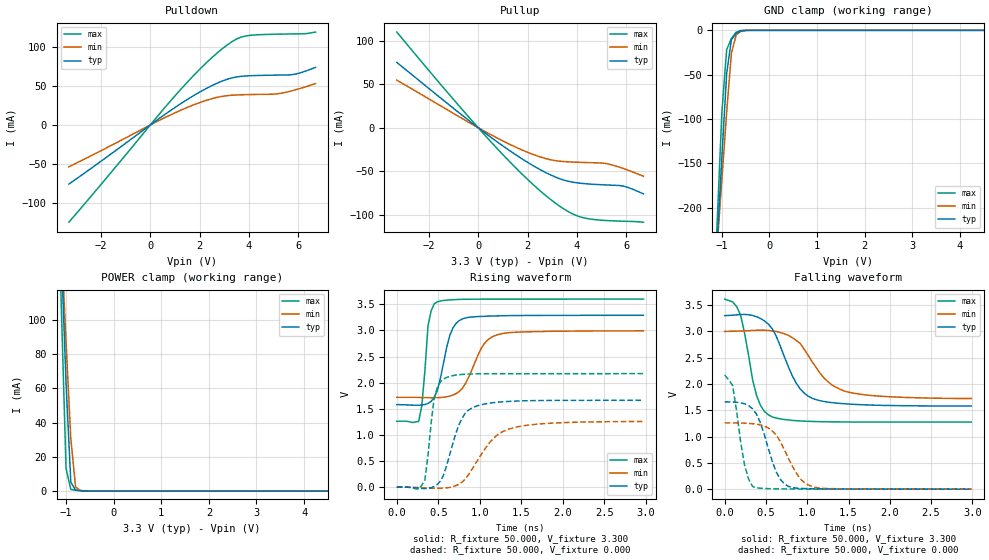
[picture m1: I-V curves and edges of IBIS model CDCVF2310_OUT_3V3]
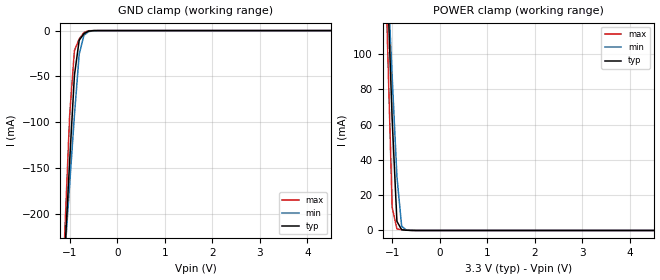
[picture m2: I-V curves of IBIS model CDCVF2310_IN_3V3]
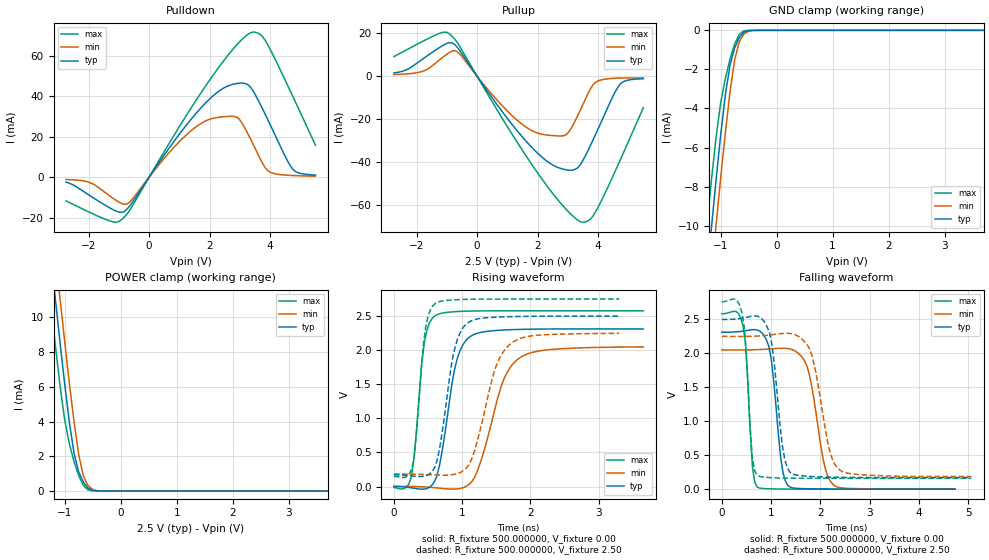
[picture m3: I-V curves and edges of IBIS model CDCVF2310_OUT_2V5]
|   TEXAS INSTRUMENTS INCORPORATED
|   CLOCK DISTRIBUTION CIRCUITS
|   IBIS Model of CDCVF2310
|   2.5-V TO 3.3-V High Performance Clock Buffer
|   24-pin (PW) Package
[IBIS Ver]   3.2
[File Name]   scac026c.ibs
[File Rev]   2.2 (10)
[Date]   12/15/2007
[Source]   File originated at Texas Instruments, Inc.
[Notes]   The following is an IBIS list for the CDCVF2310.
|   - All test data contained in this file are derived from
|   hspice(tm) simulations.
|   - File created by Gerd Baumann, HPA-Product Engineering.
|   07: added V-T tables,
|   08: corrected C_comp, revised clamp current
|   09: added R_load to ramp and corrected ramp rate
|   10: added Models for 2.5V VCC
|   (by Christian Schmoeller, 15-Dec-2007)
[Disclaimer] Property of Texas Instruments Incorporated.  Unauthorized
   reproduction and/or distribution is strictly prohibited.
   This product is protected under copyright law.
   Created 2000, (C) Copyright 2000, Texas Instruments Inc.,
   All Rights Reserved
   UNLESS THERE IS A SIGNED, WRITTEN AGREEMENT TO THE
   CONTRARY, TEXAS INSTRUMENTS ("TI") IS PROVIDING THE IBIS
   MODELS "AS IS" AND WITHOUT ANY WARRANTY, EXPRESSED OR
   IMPLIED.  TI assumes no liability for:
   1) the accuracy of the IBIS models provided to your
   company;
   2) the proper functioning of these IBIS models in your
   design or for any resulting applications; or
   3) infringement of patents, copyrights or intellectual
   property rights resulting from your use of these IBIS
   models.
   TI provides IBIS Models as a service to our customers.
   You and your company shall not distribute, sell or give
   these models to anyone else without prior written
   permission from TI.
   TI reserves the right to make changes to our products or
   to discontinue any semiconductor product or service
   without notice, and advises our customers to obtain the
   latest version of relevant information to verify, before
   placing orders, that the information being relied on is
   current.
   Please be aware that your receipt and use of the IBIS
   information provided shall serve as acceptance of these
   terms and conditions.  If you do not accept these terms,
   you should return or destroy the IBIS models and any
   other accompanying information immediately.
[Component]   CDCVF2310(High_Performance_Clock_Buffer)
[Manufacturer]  Texas Instruments, Inc.
[Package]
|   typ   min   max
R_pkg   0.034   0.031   0.040
L_pkg   2.71n   2.07n   3.51n
C_pkg   0.37p   0.24p   0.48p
[Pin]   signal_name   model_name   R_pin   L_pin   C_pin
 1   GND   GND   0.035   3.51n   0.48p
 2   VCC   POWER   0.040   3.26n   0.47p
 3   1Y0   CDCVF2310_OUT   0.035   2.96n   0.42p
 4   1Y1   CDCVF2310_OUT   0.031   2.33n   0.32p
 5   1Y2   CDCVF2310_OUT   0.032   2.14n   0.26p
 6   GND   GND   0.031   2.07n   0.24p
 7   GND   GND   0.031   2.07n   0.24p
 8   1Y3   CDCVF2310_OUT   0.032   2.14n   0.26p
 9   1Y4   CDCVF2310_OUT   0.031   2.33n   0.32p
10   VCC   POWER   0.035   2.96n   0.42p
11   1G   CDCVF2310_IN   0.040   3.26n   0.47p
12   2Y4   CDCVF2310_OUT   0.035   3.51n   0.48p
13   2G   CDCVF2310_IN   0.035   3.51n   0.48p
14   VCC   POWER   0.040   3.26n   0.47p
15   VCC   POWER   0.035   2.96n   0.42p
16   2Y3   CDCVF2310_OUT   0.031   2.33n   0.32p
17   2Y2   CDCVF2310_OUT   0.032   2.14n   0.26p
18   GND   GND   0.031   2.07n   0.24p
19   GND   GND   0.031   2.07n   0.24p
20   2Y1   CDCVF2310_OUT   0.032   2.14n   0.26p
21   2Y0   CDCVF2310_OUT   0.031   2.33n   0.32p
22   VCC   POWER   0.035   2.96n   0.42p
23   VCC   POWER   0.040   3.26n   0.47p
24   CLK   CDCVF2310_IN   0.035   3.51n   0.48p
[Model Selector]   CDCVF2310_IN
CDCVF2310_IN_2V5   Model for 2.5V VCC
CDCVF2310_IN_3V3   Model for 3.3V VCC
[Model Selector]   CDCVF2310_OUT
CDCVF2310_OUT_2V5   Model for 2.5V VCC
CDCVF2310_OUT_3V3   Model for 3.3V VCC
| Models and submodels in the file (4): CDCVF2310_OUT_3V3 (Output), CDCVF2310_IN_3V3 (Input), CDCVF2310_OUT_2V5 (Output), CDCVF2310_IN_2V5 (Input)
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|   Model CDCVF2510_OUT
[Model]   CDCVF2310_OUT_3V3
Model_type   Output
Polarity   Non-Inverting
Enable   Active-High
Vmeas = 1.65V   |Vref for timing measurements.
Cref = 25pF   |load capacitance for timing spec.
Rref = 500   |500 Ohm to GND.
Vref = 0   |Timing specification test load voltage; GND
| variable   typ   min   max
C_comp   2.4pF   NA   NA
[Temperature Range]   40   85   -40
[Voltage range]   3.3   3.0   3.6
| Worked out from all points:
|   slope of the pulldown table from 0 to 0.495 V, typ, clamps not added: 43.4 ohm
|   slope of the pullup table from 0 to 0.495 V, typ, clamps not added: 46.8 ohm
|   GND clamp passes 1 mA (typ) near -0.61 V on its own axis
|   POWER clamp passes 1 mA (typ) near -0.81 V on its own axis
|   rising waveform, R_fixture 50.000, V_fixture 3.300: 20-80 % time 151ps typ, 227ps min, 70.9ps max; typ from 1.58 V to 3.29 V
|   rising waveform, R_fixture 50.000, V_fixture 0.000: 20-80 % time 208ps typ, 349ps min, 92.9ps max; typ from 0 V to 1.66 V
|   falling waveform, R_fixture 50.000, V_fixture 3.300: 20-80 % time 299ps typ, 375ps min, 181ps max; typ from 3.3 V to 1.58 V
|   falling waveform, R_fixture 50.000, V_fixture 0.000: 20-80 % time 210ps typ, 257ps min, 125ps max; typ from 1.66 V to 0 V
|Process range|   nominal   weak   strong
[Pullup]
|   40C:3.3V:nominal   85C:3.0V:weak   -40C:3.6V:strong
|Voltage   I(typ)   I(min)   I(max)
-3.3V     75.19mA    54.67mA    110mA
-1.1V     24.53mA    18.06mA    35.81mA
500mV     -10.69mA   -7.798mA   -15.73mA
1.9V      -38.04mA   -27.06mA   -56.69mA
2.9V      -53.85mA   -36.64mA   -81.76mA
3.3V      -58.62mA   -38.52mA   -90.21mA
3.7V      -61.95mA   -39.31mA   -97.27mA
4.3V      -64.28mA   -39.98mA   -103.8mA
5.1V      -65.71mA   -40.83mA   -106.6mA
5.9V      -67.24mA   -47.1mA    -107.6mA
6.7V      -76.07mA   -55.82mA   -108.6mA
[Pulldown]
|   40C:3.3V:nominal   85C:3.0V:weak   -40C:3.6V:strong
|   Voltage   I(typ)   I(min)   I(max)
-3.3V     -76.04mA   -53.76mA   -125mA
1.1V      24.61mA    17.09mA    41.07mA
2.1V      44.08mA    29.92mA    74.72mA
2.7V      53.67mA    35.49mA    92.38mA
3.1V      58.67mA    37.69mA    102.6mA
3.5V      61.85mA    38.64mA    110.7mA
3.9V      63.13mA    39.07mA    114.7mA
5.1V      64.18mA    39.88mA    116.8mA
5.7V      64.55mA    43.63mA    117.1mA
6.3V      69.38mA    49.18mA    117.4mA
6.7V      74.16mA    53.29mA    119.5mA
[GND CLAMP]
|   40C:3.3V:nominal   85C:3.0V:weak   -40C:3.6V:strong
|   Voltage   I(typ)   I(min)   I(max)
-3.6V     -2.711A    -2.15A     -3.417A
-1.2V     -339.5mA   -320.2mA   -345.4mA
-1.1V     -240.7mA   -244mA     -217.5mA
-1V       -142.4mA   -167.9mA   -92.25mA
-900mV    -48.93mA   -92.6mA    -21.84mA
-800mV    -10.62mA   -25.94mA   -9.2mA
-700mV    -3.38mA    -5.012mA   -2.1mA
-600mV    -584.9uA   -1.132mA   -168.9uA
-400mV    -2.829uA   -16.92uA   -75.06nA
6.6V      158.6pA    496.2pA    154.8pA
[POWER CLAMP]
|   40C:3.3V:nominal   85C:3.0V:weak   -40C:3.6V:strong
|   Voltage   I(typ)   I(min)   I(max)
-3.6V     2.062A     1.625A     2.608A
-1.2V     216.4mA    205.4mA    208.3mA
-1.1V     139.5mA    146.2mA    108.3mA
-1V       63.07mA    87.18mA    13.12mA
-900mV    5.167mA    30.47mA    874.7uA
-800mV    396uA      2.327mA    462.6uA
-700mV    140.5uA    202.1uA    209.6uA
6.9V      -92.2pA    -171.3pA   -82.8pA
[ramp]
| variable   typ   min   max
|dV/dt_r  1.8112/3.9335E-10   1.5967E+00/7.6225E-10   2.0318/1.5620E-10
|dV/dt_f  1.8117/5.3947E-10   1.5967E+00/8.2198E-10   2.0318/2.7385E-10
dV/dt_r   0.9960/2.1460E-10   0.7560/3.6181E-10   1.3020/9.8334E-11
dV/dt_f   1.0320/3.0776E-10   0.7680/3.9002E-10   1.4040/1.8223E-10
R_load = 50ohms
[Rising Waveform]
R_fixture = 50.000
V_fixture = 3.300
V_fixture_min = 3.000
V_fixture_max = 3.600
|  time   V(typ)   V(min)   V(max)
0s        1.58V      1.72V      1.262V
263.2ps   1.569V     1.718V     1.257V
300.8ps   1.572V     1.716V     1.553V
376ps     1.603V     1.713V     3.09V
488.8ps   1.859V     1.714V     3.546V
639.2ps   2.908V     1.743V     3.584V
789.6ps   3.219V     1.893V     3.595V
1.015ns   3.268V     2.653V     3.598V
1.203ns   3.278V     2.913V     3.599V
2.97ns    3.289V     2.992V     3.6V
[Rising Waveform]
R_fixture = 50.000
V_fixture = 0.000
|  time   V(typ)   V(min)   V(max)
0s        108.2uV    135.6uV    85.13uV
263.2ps   -18.41mV   -6.661mV   -37.71mV
338.4ps   -26.35mV   -11.53mV   138.6mV
451.2ps   14.56mV    -20.15mV   1.72V
601.6ps   421.9mV    -12.44mV   2.1V
789.6ps   1.326V     102mV      2.158V
977.6ps   1.561V     527.8mV    2.17V
1.203ns   1.624V     990mV      2.172V
1.429ns   1.647V     1.146V     2.172V
2.97ns    1.663V     1.257V     2.173V
[Falling Waveform]
R_fixture = 50.000
V_fixture = 3.300
V_fixture_min = 3.000
V_fixture_max = 3.600
|  time   V(typ)   V(min)   V(max)
0s        3.3V       3V         3.615V
192.8ps   3.321V     3.008V     3.308V
385.6ps   3.28V      3.022V     1.785V
482ps     3.199V     3.022V     1.477V
578.4ps   3.044V     3.008V     1.372V
867.6ps   2.013V     2.829V     1.303V
1.06ns    1.728V     2.422V     1.288V
1.253ns   1.655V     2.039V     1.281V
1.494ns   1.619V     1.847V     1.278V
2.988ns   1.581V     1.725V     1.276V
[Falling Waveform]
R_fixture = 50.000
V_fixture = 0.000
|  time   V(typ)   V(min)   V(max)
0s        1.66V      1.261V     2.17V
96.4ps    1.657V     1.261V     1.972V
241ps     1.624V     1.255V     452.7mV
337.4ps   1.529V     1.244V     51.2mV
433.8ps   1.256V     1.222V     17.3mV
626.6ps   321.5mV    1.03V      6.9mV
771.2ps   54mV       588.5mV    4.2mV
915.8ps   15.1mV     194.4mV    2.8mV
1.109ns   7.8mV      31.4mV     1.8mV
2.988ns   500uV      800uV      400uV
[Model]   CDCVF2310_IN_3V3
Model_type   Input
Polarity   Non-Inverting
Vinl = 0.8V
Vinh = 2.0V
| variable   typ   min   max
C_comp   2.0pF   NA   NA
[Temperature Range]   40   85   -40
[Voltage range]   3.3   3.0   3.6
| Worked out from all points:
|   GND clamp passes 1 mA (typ) near -0.61 V on its own axis
|   POWER clamp passes 1 mA (typ) near -0.81 V on its own axis
|Process range|   nominal   weak   strong
[GND CLAMP]
|   40C:3.3V:nominal   85C:3.0V:weak   -40C:3.6V:strong
|   Voltage   I(typ)   I(min)   I(max)
-3.6V     -2.711A    -2.15A     -3.417A
-1.2V     -339.5mA   -320.2mA   -345.4mA
-1.1V     -240.7mA   -244mA     -217.5mA
-1V       -142.4mA   -167.9mA   -92.25mA
-900mV    -48.93mA   -92.6mA    -21.84mA
-800mV    -10.62mA   -25.94mA   -9.2mA
-700mV    -3.38mA    -5.012mA   -2.1mA
-600mV    -584.9uA   -1.132mA   -168.9uA
-400mV    -2.829uA   -16.92uA   -75.06nA
6.6V      158.6pA    496.2pA    154.8pA
[POWER CLAMP]
|   40C:3.3V:nominal   85C:3.0V:weak   -40C:3.6V:strong
|   Voltage   I(typ)   I(min)   I(max)
-3.6V     2.062A     1.625A     2.608A
-1.2V     216.4mA    205.4mA    208.3mA
-1.1V     139.5mA    146.2mA    108.3mA
-1V       63.07mA    87.18mA    13.12mA
-900mV    5.167mA    30.47mA    874.7uA
-800mV    396uA      2.327mA    462.6uA
-700mV    140.5uA    202.1uA    209.6uA
6.9V      -92.2pA    -171.3pA   -82.8pA
[Model] CDCVF2310_OUT_2V5
| Variable   Typ   Min   Max
Model_type   Output
Polarity   Non-Inverting
Enable   Active-High
Vmeas = 1.25V   |Vref for timing measurements.
Cref = 25pF   |load capacitance for timing spec.
Rref = 500   |500 Ohm to GND.
Vref = 0   |Timing specification test load voltage; GND
| variable   typ   min   max
C_comp   2.4pF   NA   NA
|C_comp   1.788908e-12   1.740318e-12   1.834283e-12   |simulated
[Temperature range]   27   85   -40
[Voltage range]   2.500000   2.250000   2.750000
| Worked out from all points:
|   slope of the pulldown table from 0 to 0.375 V, typ, clamps not added: 45.2 ohm
|   slope of the pullup table from 0 to 0.375 V, typ, clamps not added: 49.3 ohm
|   GND clamp passes 1 mA (typ) near -0.76 V on its own axis
|   POWER clamp passes 1 mA (typ) near -0.74 V on its own axis
|   rising waveform, R_fixture 500.000000, V_fixture 0.00: 20-80 % time 224ps typ, 356ps min, 137ps max; typ from 0.002 V to 2.31 V
|   rising waveform, R_fixture 500.000000, V_fixture 2.50: 20-80 % time 212ps typ, 325ps min, 131ps max; typ from 0.172 V to 2.5 V
|   falling waveform, R_fixture 500.000000, V_fixture 0.00: 20-80 % time 181ps typ, 277ps min, 119ps max; typ from 2.31 V to 0 V
|   falling waveform, R_fixture 500.000000, V_fixture 2.50: 20-80 % time 195ps typ, 306ps min, 126ps max; typ from 2.5 V to 0.17 V
[GND Clamp]
|   Voltage   I(typ)   I(min)   I(max)
-2.75V    -61.11mA   -63.4mA    -58.62mA
-1.25V    -12.74mA   -15.16mA   -10.2mA
-1.167V   -10.21mA   -12.59mA   -7.769mA
-1.083V   -7.744mA   -10.07mA   -5.54mA
-1V       -5.415mA   -7.625mA   -3.747mA
-916.7mV  -3.35mA    -5.299mA   -2.488mA
-833.3mV  -1.815mA   -3.195mA   -1.501mA
-750mV    -912.4uA   -1.538mA   -712.7uA
-666.7mV  -371.1uA   -586.5uA   -207.8uA
-583.3mV  -94.42uA   -182.5uA   -28.68uA
-333.3mV  -139.7nA   -948nA     -4.154nA
5.5V      1.851pA    68.82pA    10.78fA
[POWER Clamp]
|   Voltage   I(typ)   I(min)   I(max)
-2.75V    62.16mA    64.7mA     59.4mA
-1.333V   16.2mA     18.81mA    13.41mA
-1.25V    13.6mA     16.2mA     10.84mA
-1.167V   11.04mA    13.61mA    8.367mA
-1.083V   8.537mA    11.07mA    6.051mA
-1V       6.141mA    8.586mA    4.086mA
-833.3mV  2.168mA    3.978mA    1.688mA
-750mV    1.088mA    2.093mA    878.6uA
-666.7mV  497.7uA    851uA      312uA
-583.3mV  162uA      296uA      57.96uA
-333.3mV  301.7nA    1.893uA    10.71nA
5.5V      -166.9pA   -5.819nA   -1.499pA
[Pulldown]
|   Voltage   I(typ)   I(min)   I(max)
-2.75V    -2.492mA   -1.189mA   -11.74mA
-1.917V   -9.577mA   -2.943mA   -17.79mA
-916.7mV  -17.46mA   -12.99mA   -21.09mA
-666.7mV  -14.75mA   -12.66mA   -16.95mA
916.7mV   19.63mA    16.31mA    23.01mA
1.917V    37.5mA     28.17mA    46.24mA
2.917V    46.42mA    29.51mA    65.84mA
3.417V    43.24mA    17mA       71.86mA
3.667V    36.34mA    9.338mA    70.78mA
3.917V    28.7mA     3.308mA    65.72mA
4.75V     3.938mA    809.7uA    40.07mA
5.5V      1.011mA    493.9uA    15.82mA
[Pullup]
|   Voltage   I(typ)   I(min)   I(max)
-2.75V    1.527mA    768.1uA    9.138mA
-1.75V    8.461mA    2.53mA     16.55mA
-916.7mV  15.61mA    11mA       19.73mA
-583.3mV  12.17mA    10.49mA    14.14mA
916.7mV   -18.04mA   -14.97mA   -21.51mA
1.917V    -34.61mA   -25.99mA   -43.19mA
2.917V    -43.41mA   -27.39mA   -61.45mA
3.417V    -41.11mA   -15.71mA   -67.62mA
3.667V    -34.6mA    -8.179mA   -67.25mA
3.917V    -27.14mA   -2.86mA    -63.13mA
4.667V    -4.891mA   -884.7uA   -41.09mA
5.5V      -1.173mA   -810.8uA   -14.58mA
[Ramp]
|  Variable  typ   min   max
dV/dt_r   1.433/2.345587e-10   1.267/3.704865e-10   1.593/1.399425e-10
dV/dt_f   1.433/2.345587e-10   1.267/3.704865e-10   1.593/1.399425e-10
R_load = 500.000000
[Rising waveform]
R_fixture = 500.000000
C_fixture = 0
L_fixture = 0
V_fixture = 0.00
V_fixture_min = 0.00
V_fixture_max = 0.00
|   Time   V(typ)   V(min)   V(max)
0s        2.341mV    1.213mV    -12.9mV
258.6ps   -19.46mV   1.567mV    154.7mV
443.4ps   -36.99mV   -4.794mV   2.094V
591.2ps   67.33mV    -16.12mV   2.497V
702ps     489.3mV    -26.95mV   2.543V
886.7ps   1.707V     -36.65mV   2.564V
1.108ns   2.193V     36.8mV     2.574V
1.589ns   2.295V     1.516V     2.577V
1.81ns    2.304V     1.863V     2.578V
3.658ns   2.312V     2.048V     2.577V
[Rising waveform]
R_fixture = 500.000000
C_fixture = 0
L_fixture = 0
V_fixture = 2.50
V_fixture_min = 2.25
V_fixture_max = 2.75
|   Time   V(typ)   V(min)   V(max)
0s        172mV      182.5mV    152.5mV
266.9ps   156.3mV    182mV      277.5mV
333.7ps   150mV      180.5mV    807.9mV
433.8ps   149.9mV    177.2mV    2.103V
600.6ps   284.7mV    170.2mV    2.681V
867.5ps   1.92V      175.4mV    2.738V
1.068ns   2.388V     275.7mV    2.746V
1.501ns   2.485V     1.773V     2.75V
1.702ns   2.492V     2.087V     2.75V
3.303ns   2.5V       2.248V     2.75V
[Falling waveform]
R_fixture = 500.000000
C_fixture = 0
L_fixture = 0
V_fixture = 0.00
V_fixture_min = 0.00
V_fixture_max = 0.00
|   Time   V(typ)   V(min)   V(max)
0s        2.311V     2.05V      2.58V
430.1ps   2.327V     2.049V     2.41V
621.3ps   2.347V     2.051V     333.5mV
716.8ps   2.343V     2.054V     32.72mV
955.8ps   2.1V       2.064V     5.741mV
1.195ns   464.4mV    2.074V     2.265mV
1.338ns   58.27mV    2.07V      1.329mV
1.72ns    6.381mV    1.825V     272.3uV
2.246ns   1.849mV    78.06mV    5.031uV
4.731ns   3.96uV     939uV      -1.078uV
[Falling waveform]
R_fixture = 500.000000
C_fixture = 0
L_fixture = 0
V_fixture = 2.50
V_fixture_min = 2.25
V_fixture_max = 2.75
|   Time   V(typ)   V(min)   V(max)
0s        2.498V     2.25V      2.755V
409.2ps   2.517V     2.248V     2.591V
613.8ps   2.548V     2.251V     500.2mV
716.1ps   2.548V     2.254V     206.2mV
971.9ps   2.295V     2.27V      170.3mV
1.228ns   642.8mV    2.292V     163.5mV
1.381ns   252.2mV    2.292V     161.7mV
1.79ns    187.2mV    2.052V     159.9mV
2.404ns   174.2mV    276.2mV    159.5mV
5.064ns   170.2mV    186.3mV    159.5mV
